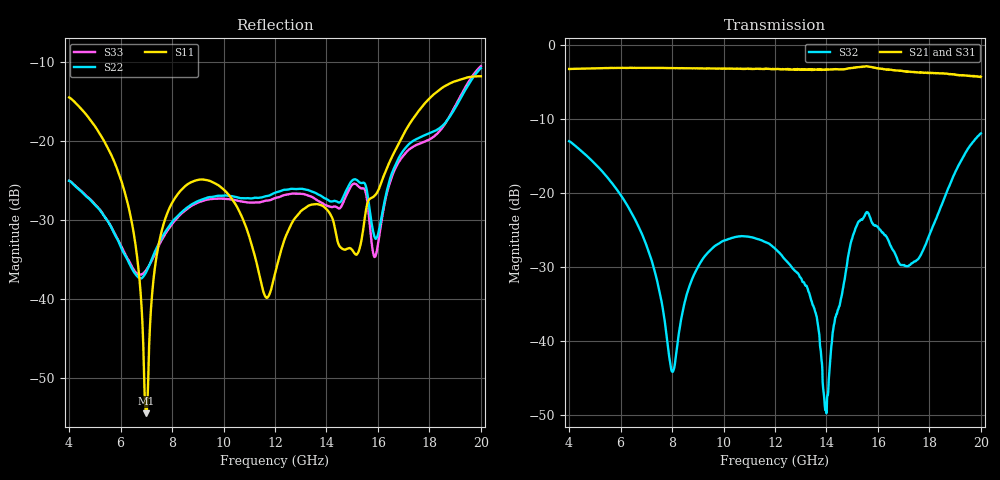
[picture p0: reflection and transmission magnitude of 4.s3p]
!The following data was pulled from an Agilent PNA
!This sNp file was generated from the data in the RF Test software
!NOTE:  Smoothing/Math/Corrections applied on any given trace ARE included in the data saved here
# MHz S dB R 50
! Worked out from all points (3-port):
!   1601 points, 4 GHz to 20 GHz, reference 50 ohm
!   strongest paths, dB at 4 GHz, 8 GHz, 12 GHz, 16 GHz, 20 GHz:
!     S21: -3.3, -3.2, -3.3, -3.2, -4.3
!     S31: -3.3, -3.2, -3.3, -3.2, -4.4
!     S32: -13.1, -44.2, -27.6, -24.6, -12.0
!   lowest |S11| = -54.5 dB at 7 GHz (marker M1), VSWR 1.00, Z = 50 - j0.187 ohm
!   |S11| at or under -10 dB: start of sweep to end of sweep
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4000  -14.47 89.8  -3.30 -108.8  -3.30 -109.2
      -3.29 -108.7  -25.06 -57.6  -13.06 -138.0
      -3.30 -109.1  -13.06 -138.0  -25.03 -57.9
6240  -27.44 31.8  -3.14 -173.7  -3.15 -174.3
      -3.15 -173.6  -34.89 -117.0  -21.62 162.2
      -3.15 -174.2  -21.61 162.2  -34.73 -118.1
7000  -54.53 -86.9  -3.15 163.5  -3.16 162.9
      -3.15 163.6  -36.58 -76.7  -27.10 144.4
      -3.16 163.0  -27.08 144.4  -36.35 -81.7
7430  -33.99 -178.2  -3.15 150.5  -3.17 149.8
      -3.16 150.5  -33.36 -64.3  -32.11 138.5
      -3.16 149.9  -32.09 138.6  -33.62 -68.0
8420  -25.99 151.6  -3.18 120.3  -3.19 119.5
      -3.19 120.2  -28.89 -70.8  -35.95 -109.5
      -3.20 119.5  -35.95 -109.5  -29.03 -72.9
12000  -36.83 -97.2  -3.29 4.3  -3.32 3.2
       -3.31 4.5  -26.56 -88.5  -27.57 164.3
       -3.30 3.5  -27.56 164.3  -27.25 -90.0
13980  -28.56 124.2  -3.36 -65.3  -3.39 -66.5
       -3.40 -65.4  -27.32 -95.1  -49.36 33.3
       -3.39 -66.6  -49.46 32.9  -28.16 -94.7
15200  -34.31 -134.4  -3.08 -111.8  -3.05 -113.4
       -3.06 -111.7  -25.00 -93.3  -24.27 -125.3
       -3.05 -113.3  -24.27 -125.2  -25.62 -94.6
16820  -20.25 -36.8  -3.49 178.9  -3.50 177.5
       -3.54 179.1  -22.08 -69.1  -29.45 170.0
       -3.59 177.5  -29.50 170.0  -22.60 -69.6
20000  -11.79 157.6  -4.53 38.3  -4.51 36.4
       -4.34 37.8  -10.76 35.2  -11.97 158.1
       -4.36 36.0  -12.01 158.4  -10.51 32.6
